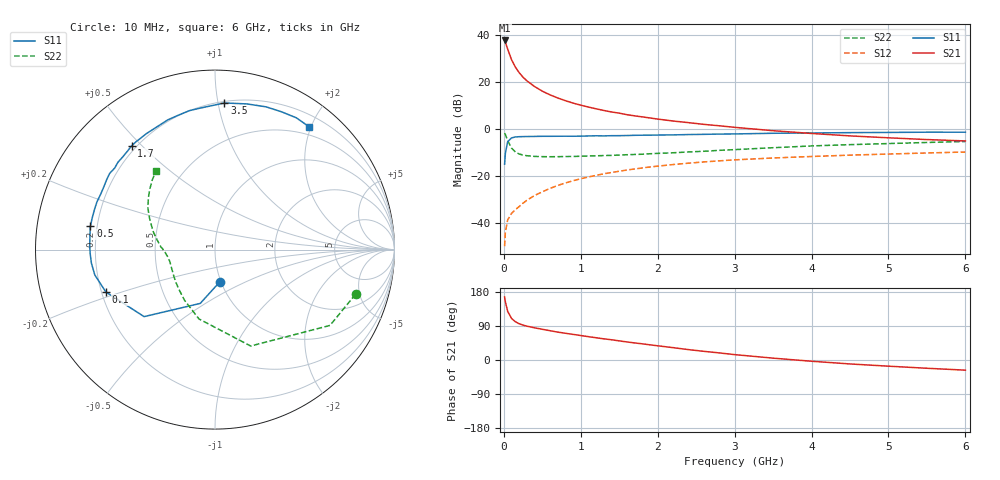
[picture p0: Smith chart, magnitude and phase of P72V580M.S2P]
! SIEMENS Small Signal Semiconductors
! BFP196
! Si NPN RF Bipolar Junction Transistor in SOT143
! VCE = 2.5 V  IC = 80 mA
! Common Emitter S-Parameters:  May  1996
# GHz  S  MA  R  50
!  f  S11  S21  S12  S22
! GHz  MAG  ANG  MAG  ANG  MAG  ANG  MAG  ANG
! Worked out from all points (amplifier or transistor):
!   36 points, 10 MHz to 6 GHz, reference 50 ohm
!   highest |S21| = 37.6 dB at 10 MHz (marker M1)
!   |S21| within 3 dB of that: start of sweep to 43.03 MHz
!   unconditionally stable (mu >= 1): 337.8 MHz to 4.547 GHz
!   at 250 MHz: K = 0.94, MSG = 26.7 dB, |S12| = -31.4 dB
!   at 1.4 GHz: K = 1.09, MAG = 11.0 dB, |S12| = -18.4 dB
!   at 6 GHz: K = 0.99, MSG = 2.4 dB, |S12| = -9.7 dB
!   S11 on the Smith chart (normalised r, x): 10 MHz: 0.99, -0.37; 100 MHz: 0.22, -0.18; 500 MHz: 0.17, +0.09; 1.7 GHz: 0.18, +0.47; 3.5 GHz: 0.21, +1.04; 6 GHz: 0.37, +1.96
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0.01  0.1812 -81.4  76.16 166.4  0.0033 76.6  0.8219 -17.6
0.02  0.3107 -105.3  69.77 153.3  0.0066 70.2  0.7673 -33.4
0.05  0.5435 -136.6  49.87 128.3  0.0119 54.0  0.5728 -69.7
0.1  0.6524 -158.8  29.81 109.6  0.0164 52.0  0.3966 -103.0
0.15  0.6844 -168.1  20.71 100.9  0.0196 54.4  0.3289 -121.2
0.2  0.6927 -173.7  15.78 95.7  0.0229 57.1  0.2975 -133.0
0.25  0.6956 -177.9  12.62 92.0  0.027 60.4  0.2821 -141.3
0.3  0.6981 178.9  10.6 89.3  0.0311 62.5  0.2735 -146.8
0.4  0.7019 173.1  8.011 84.9  0.0392 64.8  0.2644 -154.8
0.5  0.7064 169.4  6.404 81.1  0.047 65.8  0.2614 -160.0
0.6  0.7065 165.3  5.345 77.3  0.0555 66.1  0.2604 -163.4
0.7  0.7079 161.1  4.593 73.6  0.0639 66.0  0.2609 -166.0
0.9  0.7079 154.2  3.577 67.6  0.0807 64.1  0.2635 -170.1
1.1  0.7181 147.3  2.944 61.5  0.0968 62.0  0.27 -173.0
1.3  0.7202 140.9  2.496 55.8  0.1132 59.3  0.2755 -175.7
1.7  0.7414 128.8  1.917 45.0  0.1431 53.6  0.2908 179.4
2.2  0.7563 115.5  1.49 32.6  0.1778 45.7  0.3159 173.2
2.8  0.7872 100.4  1.18 18.7  0.2129 36.5  0.3556 164.4
3.5  0.8187 86.3  0.928 4.9  0.2449 26.4  0.4045 154.4
4.5  0.8448 70.3  0.72 -10.4  0.2814 14.3  0.4698 142.2
5.5  0.8629 58.3  0.602 -21.8  0.3129 3.4  0.5223 132.0
6  0.8621 52.7  0.563 -26.8  0.3277 -2.3  0.5474 126.9
